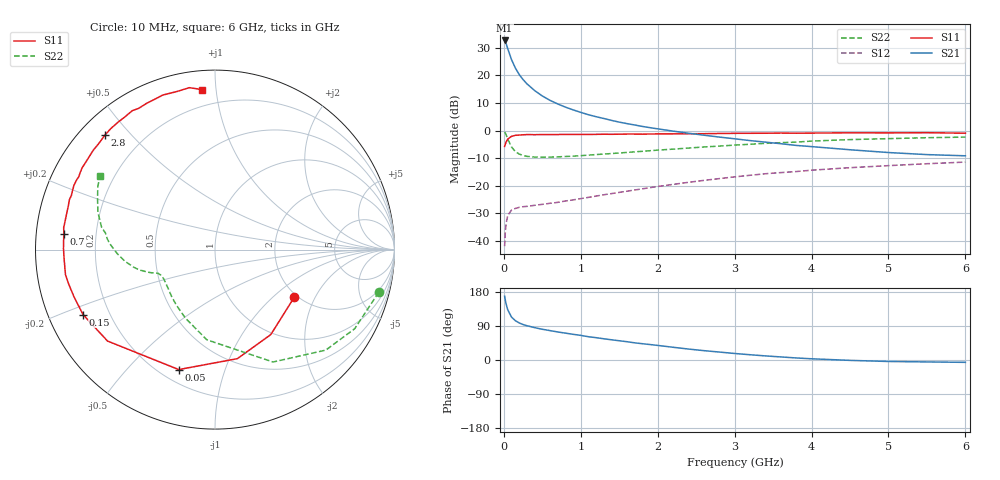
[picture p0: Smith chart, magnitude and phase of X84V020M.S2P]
! SIEMENS Small Signal Semiconductors
! BFP136W
! Si NPN RF Bipolar Junction Transistor in SOT343
! VCE = 4 V  IC = 20 mA
! Common Emitter S-Parameters:  September  1994
# GHz  S  MA  R  50
!  f  S11  S21  S12  S22
! GHz  MAG  ANG  MAG  ANG  MAG  ANG  MAG  ANG
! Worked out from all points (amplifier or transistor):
!   40 points, 10 MHz to 6 GHz, reference 50 ohm
!   highest |S21| = 32.6 dB at 10 MHz (marker M1)
!   |S21| within 3 dB of that: start of sweep to 51.15 MHz
!   unconditionally stable (mu >= 1): 875.8 MHz to 2.76 GHz
!   at 200 MHz: K = 0.33, MSG = 24.0 dB, |S12| = -27.8 dB
!   at 1.5 GHz: K = 1.16, MAG = 10.3 dB, |S12| = -22.4 dB
!   at 6 GHz: K = 0.98, MSG = 1.1 dB, |S12| = -11.4 dB
!   S11 on the Smith chart (normalised r, x): 10 MHz: 1.93, -1.39; 50 MHz: 0.27, -0.71; 150 MHz: 0.10, -0.23; 700 MHz: 0.08, +0.05; 2.8 GHz: 0.07, +0.42; 6 GHz: 0.10, +0.92
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0.01  0.5153 -30.8  42.58 168.3  0.0081 76.4  0.943 -14.6
0.02  0.5664 -56.7  39.81 157.1  0.0152 68.3  0.8945 -29.5
0.03  0.6203 -78.4  37.25 147.7  0.0209 60.4  0.8335 -42.2
0.05  0.6982 -106.8  30.47 132.8  0.0289 46.5  0.7048 -62.7
0.1  0.7862 -139.6  19.13 113.2  0.0365 31.3  0.5044 -95.2
0.15  0.8196 -153.8  13.5 103.7  0.039 26.6  0.4157 -113.4
0.2  0.8286 -161.6  10.28 97.8  0.0408 24.7  0.3756 -125.3
0.25  0.8378 -166.9  8.344 93.6  0.0419 24.5  0.3543 -133.4
0.3  0.8447 -170.5  7.003 90.5  0.0425 24.6  0.3413 -139.0
0.4  0.8421 -176.2  5.286 85.4  0.0444 26.6  0.3315 -146.4
0.5  0.8442 179.7  4.221 81.1  0.0462 28.8  0.3291 -150.8
0.6  0.8448 177.0  3.515 77.6  0.0483 31.6  0.3307 -153.4
0.7  0.8467 174.0  3.03 74.0  0.0502 34.4  0.3341 -155.0
0.9  0.8501 169.6  2.365 67.8  0.0556 38.8  0.3439 -157.5
1.1  0.8513 164.9  1.931 61.4  0.0618 42.7  0.3592 -158.7
1.5  0.8585 157.8  1.42 50.8  0.076 48.5  0.3925 -161.3
2.2  0.8699 144.9  0.976 33.6  0.1061 51.5  0.4609 -167.5
2.8  0.8849 133.9  0.762 21.0  0.135 49.9  0.5233 -175.0
3.2  0.892 127.3  0.658 13.9  0.155 47.3  0.5645 179.6
4.5  0.9089 108.6  0.449 -1.0  0.2129 36.3  0.6854 162.2
5.5  0.9134 99.0  0.367 -5.1  0.2509 27.9  0.7417 151.7
6  0.8947 94.7  0.349 -6.2  0.2688 23.4  0.7607 147.3
